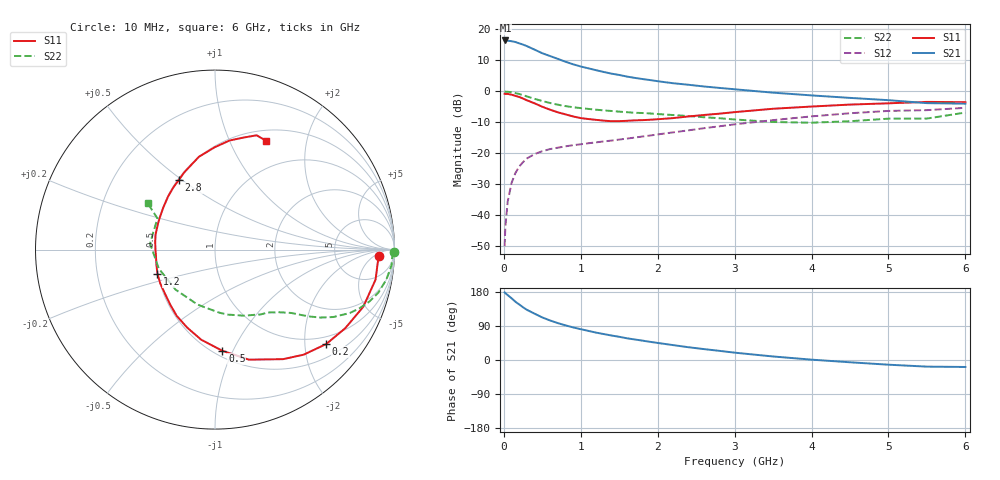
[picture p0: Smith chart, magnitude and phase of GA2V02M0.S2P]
! Infineon Technologies  Discrete & RF Semiconductors
! BF775
! Si NPN RF Bipolar Junction Transistor in SOT23
! VCE = 2 V  IC = 2 mA
! Common Emitter S-Parameters:  May  1996
# GHz  S  MA  R  50
!  f  S11  S21  S12  S22
! GHz  MAG  ANG  MAG  ANG  MAG  ANG  MAG  ANG
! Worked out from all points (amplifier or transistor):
!   36 points, 10 MHz to 6 GHz, reference 50 ohm
!   highest |S21| = 16.4 dB at 20 MHz (marker M1)
!   |S21| within 3 dB of that: start of sweep to 403 MHz
!   unconditionally stable (mu >= 1): 1.145 GHz to 4.364 GHz; 5.034 GHz to end of sweep
!   at 250 MHz: K = 0.29, MSG = 18.9 dB, |S12| = -22.8 dB
!   at 1.4 GHz: K = 1.12, MAG = 8.7 dB, |S12| = -15.9 dB
!   at 6 GHz: K = 1.02, MAG = -0.3 dB, |S12| = -5.3 dB
!   S11 on the Smith chart (normalised r, x): 10 MHz: 19, -8; 200 MHz: 0.81, -2.50; 500 MHz: 0.55, -0.91; 1.2 GHz: 0.50, -0.15; 2.8 GHz: 0.51, +0.49; 6 GHz: 0.63, +1.38
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0.01  0.9156 -2.2  6.558 178.5  0.0032 89.0  0.9979 -0.9
0.02  0.91 -4.2  6.625 176.3  0.0066 86.0  0.9885 -2.0
0.05  0.9101 -10.6  6.568 171.3  0.0167 82.6  0.9874 -5.1
0.1  0.8853 -21.1  6.442 163.0  0.0334 77.7  0.9688 -10.0
0.15  0.8476 -31.1  6.253 153.8  0.0482 71.9  0.9411 -14.8
0.2  0.813 -40.3  5.953 146.5  0.0616 66.9  0.9075 -18.6
0.25  0.7662 -49.8  5.678 139.1  0.0726 62.0  0.869 -22.1
0.3  0.7189 -58.1  5.367 132.4  0.083 59.0  0.83 -25.2
0.4  0.6416 -72.9  4.709 122.2  0.0977 52.9  0.7582 -29.7
0.5  0.5654 -85.8  4.123 112.3  0.1087 48.5  0.6989 -32.8
0.6  0.5076 -98.8  3.716 104.4  0.1175 45.6  0.6509 -35.0
0.7  0.461 -109.7  3.351 97.5  0.1236 43.8  0.6111 -36.8
0.8  0.4265 -120.0  3.012 91.5  0.1301 42.6  0.5796 -38.3
1.1  0.3584 -148.4  2.352 76.8  0.146 41.4  0.5219 -42.2
1.2  0.3478 -157.2  2.195 72.2  0.1509 41.3  0.5073 -43.6
1.6  0.3357 173.0  1.734 57.3  0.1735 43.0  0.462 -49.3
2.2  0.3712 140.9  1.354 39.3  0.2185 44.0  0.4157 -61.5
2.8  0.4373 117.4  1.139 24.2  0.2737 41.9  0.3696 -78.7
3.5  0.5251 99.8  0.954 9.3  0.3442 36.0  0.3215 -107.6
4.5  0.6131 82.4  0.786 -6.0  0.4445 23.7  0.3306 -161.4
5.5  0.6777 70.0  0.647 -17.5  0.4987 8.4  0.365 151.5
6  0.6698 64.7  0.634 -18.4  0.5437 4.1  0.4562 145.4
